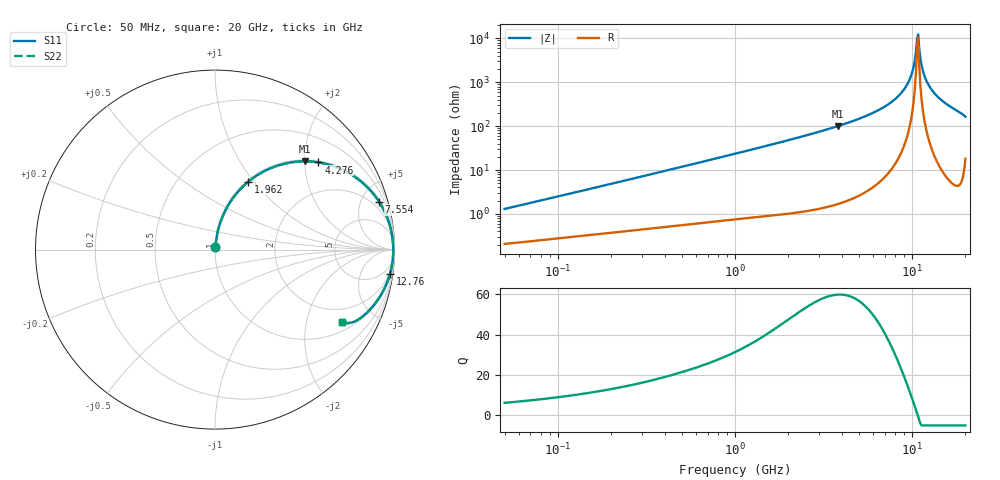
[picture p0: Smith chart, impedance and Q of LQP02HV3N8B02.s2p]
!Murata Part Number: LQP02HV3N8B02
!These Parameters are Measured in Series Mode Connection
!  o--[Z]--o
!Port1  Port2
!  o-------o
!Freq. Start=50[MHz] Stop=20[GHz], 401[Steps]
# Hz S RI R 50
!Freq.(Hz) S11(Real) S11(Imag) S21(Real) S21(Imag) S12(Real) S12(Imag) S22(Real) S22(Imag)
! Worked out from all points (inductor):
!   401 points, 50 MHz to 20 GHz, reference 50 ohm
!   read as one part in series: L = 4.03 nH near 51.52 MHz
!   highest Q = 59.9 at 3.793 GHz (marker M1), where L = 4.19 nH
!   self-resonance near 10.66 GHz
!   S11 on the Smith chart (normalised r, x): 50 MHz: 1.00, +0.03; 1.962 GHz: 1.02, +0.94; 4.276 GHz: 1.04, +2.34; 7.554 GHz: 1.20, +6.84; 12.76 GHz: 2, -14; 20 GHz: 1.36, -3.26
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5e7  0.00223 0.0128  0.9978 -0.0128  0.9978 -0.0128  0.00223 0.0128
1.364002e8  0.00425 0.0332  0.9958 -0.0332  0.9958 -0.0332  0.00425 0.0332
3.721004e8  0.0125 0.0869  0.9875 -0.0869  0.9875 -0.0869  0.0125 0.0869
1e9  0.0586 0.2195  0.9414 -0.2195  0.9414 -0.2195  0.0586 0.2195
1.962148e9  0.1857 0.3784  0.8143 -0.3784  0.8143 -0.3784  0.1857 0.3784
2.728004e9  0.3148 0.4555  0.6852 -0.4555  0.6852 -0.4555  0.3148 0.4555
3.792786e9  0.4992 0.4917  0.5008 -0.4917  0.5008 -0.4917  0.4992 0.4917
4.275624e9  0.5766 0.4858  0.4234 -0.4858  0.4234 -0.4858  0.5766 0.4858
5.856089e9  0.7813 0.4037  0.2187 -0.4037  0.2187 -0.4037  0.7813 0.4037
7.442007e9  0.9086 0.2747  0.0914 -0.2747  0.0914 -0.2747  0.9086 0.2747
7.554318e9  0.915 0.265  0.085 -0.265  0.085 -0.265  0.915 0.265
8.644534e9  0.9621 0.1706  0.0379 -0.1706  0.0379 -0.1706  0.9621 0.1706
9.457416e9  0.9821 0.1024  0.0179 -0.1024  0.0179 -0.1024  0.9821 0.1024
1.004137e10  0.9898 0.0554  0.0102 -0.0554  0.0102 -0.0554  0.9898 0.0554
1.050288e10  0.9927 0.0197  0.00732 -0.0197  0.00732 -0.0197  0.9927 0.0197
1.082228e10  0.9931 -0.0042  0.00687 0.0042  0.00687 0.0042  0.9931 -0.0042
1.098561e10  0.9929 -0.0162  0.00708 0.0162  0.00708 0.0162  0.9929 -0.0162
1.131968e10  0.9916 -0.0401  0.00837 0.0401  0.00837 0.0401  0.9916 -0.0401
1.166392e10  0.9892 -0.0639  0.0108 0.0639  0.0108 0.0639  0.9892 -0.0639
1.276073e10  0.975 -0.1343  0.025 0.1343  0.025 0.1343  0.975 -0.1343
1.527346e10  0.9166 -0.2654  0.0834 0.2654  0.0834 0.2654  0.9166 -0.2654
2e10  0.7088 -0.4023  0.2912 0.4023  0.2912 0.4023  0.7088 -0.4023
